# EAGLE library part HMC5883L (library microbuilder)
HMC5883L 3-Axis Digital Compass
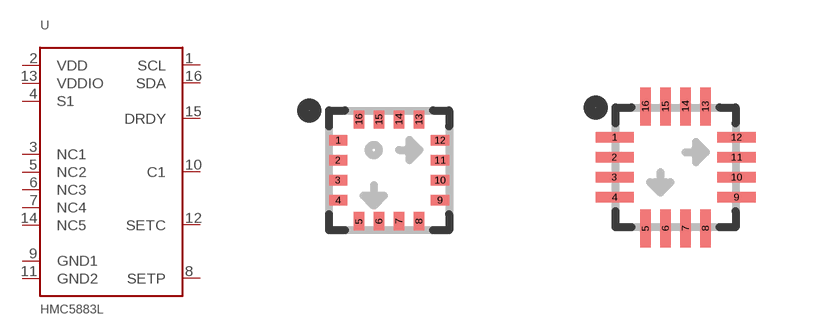
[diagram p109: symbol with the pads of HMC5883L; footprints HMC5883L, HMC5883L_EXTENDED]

Designator prefix U

## HMC5883L  [HMC5883L]
1  SCL
2  VDD
3  NC1
4  S1
5  NC2
6  NC3
7  NC4
8  SETP
9  GND1
10  C1
11  GND2
12  SETC
13  VDDIO
14  NC5
15  DRDY
16  SDA

## HMC5883LEXT  [HMC5883L_EXTENDED]
Pads as for HMC5883L

## Footprint HMC5883L (pad centres in mm)
smd 0.45 x 0.26: 1 -1.275,0.75; 2 -1.275,0.25; 3 -1.275,-0.25; 4 -1.275,-0.75; 9 1.275,-0.75; 10 1.275,-0.25; 11 1.275,0.25; 12 1.275,0.75
smd 0.26 x 0.45: 5 -0.75,-1.275; 6 -0.25,-1.275; 7 0.25,-1.275; 8 0.75,-1.275; 13 0.75,1.275; 14 0.25,1.275; 15 -0.25,1.275; 16 -0.75,1.275

## Footprint HMC5883L_EXTENDED (pad centres in mm)
smd 0.95 x 0.26: 1 -1.525,0.75; 2 -1.525,0.25; 3 -1.525,-0.25; 4 -1.525,-0.75; 9 1.525,-0.75; 10 1.525,-0.25; 11 1.525,0.25; 12 1.525,0.75
smd 0.26 x 0.95: 5 -0.75,-1.525; 6 -0.25,-1.525; 7 0.25,-1.525; 8 0.75,-1.525; 13 0.75,1.525; 14 0.25,1.525; 15 -0.25,1.525; 16 -0.75,1.525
